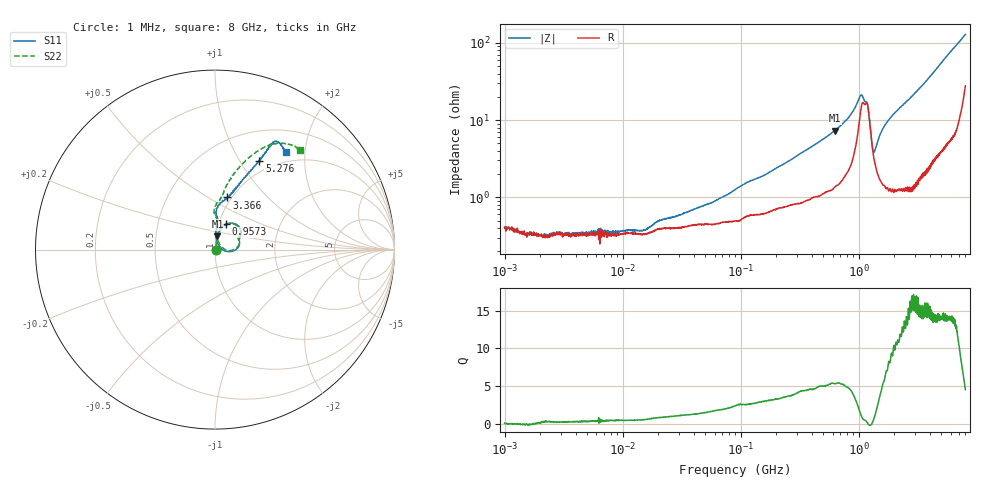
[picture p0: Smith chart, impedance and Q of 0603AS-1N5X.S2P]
!s-Parameter Generated by FASTRON Sdn. Bhd.
!FASTRON P/N : 0603AS-1N5X
!Keysight Technologies: E5071C_MY46733604_B.14.02
!Date: Tue Oct 24 10:18:28 2023
!Version  :Rev01  Tue Oct 24 10:18:28 2023
!Data & Calibration Information:
!Freq  S11:SOLT2(ON)  S21:SOLT2(ON)  S12:SOLT2(ON)  S22:SOLT2(ON)
!PortZ  Port1:50+j0  Port2:50+j0
!When reading reference impedance value at option line is always used.
! Remarks : This data is being provided solely for informational purposes.
# Hz S dB R 50
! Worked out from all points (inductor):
!   1601 points, 1 MHz to 8 GHz, reference 50 ohm
!   read as one part in series: L = 1.76 nH near 159.9 MHz
!   highest Q = 5.36 at 625.8 MHz (marker M1), where L = 1.83 nH
!   self-resonance near 1.194 GHz
!   S11 on the Smith chart (normalised r, x): 1 MHz: 1.01, -0.00; 957.3 MHz: 1.08, +0.31; 3.366 GHz: 0.95, +0.61; 5.276 GHz: 0.86, +1.22; 8 GHz: 0.84, +1.64
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1000000  -46.84 -4.2  -0.03 -0.1  -0.03 0.0  -47.05 1.8
1568286  -50.89 -18.6  -0.03 -0.0  -0.03 -0.0  -47.37 -29.5
2211112  -50.48 8.4  -0.03 -0.0  -0.03 -0.1  -53.93 33.3
2905262  -50.96 7.2  -0.04 -0.1  -0.04 -0.0  -51.75 7.3
4479405  -49.75 13.7  -0.03 -0.1  -0.04 -0.0  -51.94 21.1
8407329  -49.35 18.8  -0.03 -0.1  -0.03 -0.1  -49.94 21.5
1.552719e7  -58.87 -21.3  -0.03 -0.2  -0.04 -0.2  -46.19 21.9
2.00676e7  -47.26 36.8  -0.03 -0.2  -0.04 -0.1  -45.92 46.9
6.021717e7  -41.79 62.9  -0.04 -0.5  -0.05 -0.5  -41.58 58.3
8.994653e7  -38.21 69.2  -0.04 -0.7  -0.05 -0.7  -38.75 65.8
4.006501e8  -26.61 79.1  -0.11 -2.4  -0.12 -2.4  -26.62 78.2
6.257563e8  -22.49 79.5  -0.17 -3.8  -0.18 -3.8  -22.45 78.4
9.573479e8  -16.26 67.0  -0.60 -7.7  -0.61 -7.7  -16.29 65.2
1.041574e9  -14.64 45.6  -1.27 -7.5  -1.28 -7.5  -14.81 44.0
1.142645e9  -16.77 21.0  -1.38 -2.5  -1.39 -2.6  -16.96 24.2
1.326347e9  -30.08 44.8  -0.39 -0.2  -0.39 -0.3  -28.50 38.1
1.52743e9  -22.81 85.1  -0.26 -3.1  -0.27 -3.1  -22.79 80.9
1.7949e9  -19.37 87.8  -0.28 -5.1  -0.28 -5.2  -19.46 84.5
3.365624e9  -10.53 77.3  -0.85 -12.0  -0.85 -12.0  -10.65 83.5
5.276366e9  -5.17 63.4  -2.38 -22.6  -2.38 -22.6  -5.04 68.9
6.843354e9  -3.28 61.2  -4.56 -28.9  -4.55 -29.2  -3.13 58.4
8e9  -3.49 54.0  -6.54 -30.5  -6.53 -30.9  -2.71 49.6
